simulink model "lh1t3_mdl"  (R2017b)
settings: Solver=VariableStepDiscrete  StartTime=0.0  StopTime=10.0  RelTol=1e-3  AbsTol=1e-6
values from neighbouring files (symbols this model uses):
  A = A(1:2*N, 1:2*N)    [lh1t3_m.m]
  B = zeros(2*N, 1)    [lh1t3_m.m]
  C = eye(2*N)    [lh1t3_m.m]
  D = zeros(2*N, 1)    [lh1t3_m.m]
  x0 = 10    [lh1t4_m.m]
undefined symbols (not defined in the file or in its folder): lh1t3_suhde
libraries: simulink x1

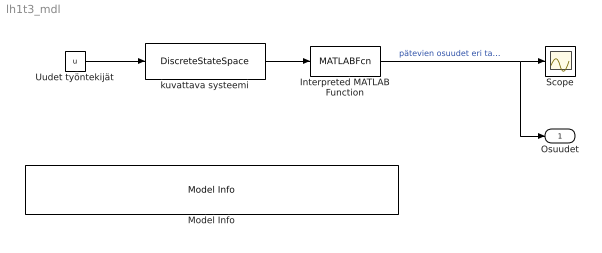
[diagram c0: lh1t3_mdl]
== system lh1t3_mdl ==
  Interpreted MATLAB Function : MATLABFcn  MATLABFcn=lh1t3_suhde(u)
  Model Info : simulink/Model-Wide Utilities/Model Info  Frame=on  DisplayStringWithTags=Laskuharjoitus 1, tehtävä 3. Alusta muuttujat ja käynnistä simulaatio ajamalla lh1t3_m.m  HorizontalTextAlignment=Center  LeftAlignmentValue=0.5
  Scope : Scope
  Uudet työntekijät : Constant  Value=u
  kuvattava systeemi : DiscreteStateSpace  A=A  B=B  C=C  D=D  InitialCondition=x0
  Osuudet : Outport
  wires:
  Interpreted MATLAB Function/1 -> Osuudet/1, Scope/1  "pätevien osuudet eri tasoilla"
  Uudet työntekijät/1 -> kuvattava systeemi/1
  kuvattava systeemi/1 -> Interpreted MATLAB Function/1
